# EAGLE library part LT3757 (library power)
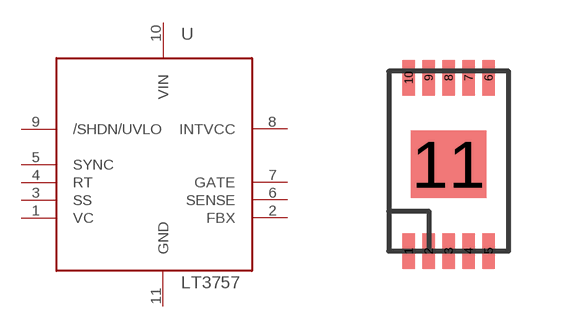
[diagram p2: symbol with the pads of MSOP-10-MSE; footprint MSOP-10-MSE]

Designator prefix U

## LT3757  [MSOP-10-MSE]
1  VC
2  FBX
3  SS
4  RT
5  SYNC
6  SENSE
7  GATE
8  INTVCC
9  /SHDN/UVLO
10  VIN
11  GND

## Footprint MSOP-10-MSE (pad centres in mm)
smd 0.305 x 0.889: 1 0,0; 2 0.5,0; 3 1,0; 4 1.5,0; 5 2,0; 6 2,4.34; 7 1.5,4.34; 8 1,4.34; 9 0.5,4.34; 10 0,4.34
smd 1.88 x 1.68: 11 1,2.17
